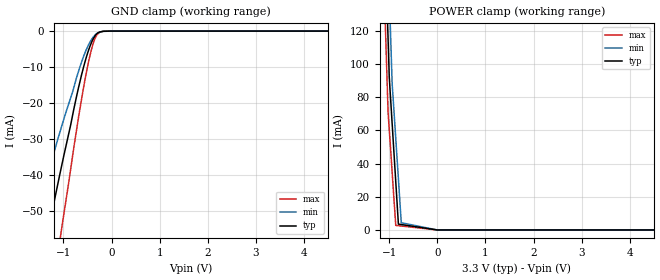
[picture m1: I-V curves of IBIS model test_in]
|DESCRIPTION OF BUG:
|Placing multiple decimal points in sequence in an IBIS file [Package]
|section causes the IBIS parser to "crash" or end execution abruptly.
|The "crash" does not occur if repeated decimal points are present in
|sections other than under the [Package] keyword.
|The parser should flag the repeated decimal points as a simple syntax
|error.
|This problem also occurs in earlier parser versions.
[IBIS Ver]   3.2
[File name]   bug59.ibs
[File rev]   1.0
[Date]   08/01/01
[Source]   From silicon level SPICE model at Intel Corporation.
[Notes]   The following information is for demo purposes only.
[Disclaimer] This IBIS model is provided in connection with Intel
   products. No license, express or implied, by estoppel or
   otherwise, to any intellectual property rights is granted
   by this document. Except as provided in Intel's Terms and
   Conditions of Sale for such products, Intel assumes no
   liability whatsoever, and Intel disclaims any express or
   implied warranty, relating to sale and/or use of Intel
   products including liability or warranties relating to
   fitness for a particular purpose, merchantability, or
   infringement of any patent, copyright or other
   intellectual property right. Intel products are not
   intended for use in medical, life saving, or life
   sustaining applications.
[Copyright]   Copyright 2001, Intel Corporation, All Rights Reserved.
[Component]   TEST
[Manufacturer]  Intel Corporation
[Package]
|   typ   min   max
R_pkg   0mOhm   0mOhm   0mOhm
L_pkg   0.00nH   0.00nH   0.00nH
C_pkg   0..00pF   0.00pF   0.00pF
[Pin]   signal_name   model_name   R_pin   L_pin   C_pin
1   TEST_IN   test_in
| Models and submodels in the file (1): test_in (Input)
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[Model]   test_in
Model_type   Input
Vinl = 0.8V
Vinh = 2.0V
|   typ   min   max
C_comp   3.11pF   2.69pF   3.33pF
[Voltage Range]   3.300V   3.135V   3.465V
[Temperature Range]   25.0   100.0   0.0
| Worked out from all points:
|   GND clamp passes 1 mA (typ) near -0.32 V on its own axis
[GND Clamp]
|   Voltage   I(typ)   I(min)   I(max)
-3.3V     -203.8mA   -150.7mA   -277.6mA
-1.725V   -84.17mA   NA         NA
-1.54V    -71.04mA   NA         NA
-1.33V    -56.54mA   NA         NA
-1.08V    -40.1mA    NA         NA
-995mV    -34.78mA   NA         NA
-695mV    -16.2mA    NA         NA
-495mV    -6.008mA   NA         NA
-375mV    -2.013mA   NA         NA
-315mV    -878.5uA   NA         NA
-250mV    -273.8uA   NA         NA
6.595V    0A         0A         0A
[POWER Clamp]
|   Voltage   I(typ)   I(min)   I(max)
-3.3V     2.388A     2.407A     2.381A
-2.055V   1.081A     NA         NA
-1V       92.25mA    NA         NA
-810mV    3.539mA    NA         NA
0V        1.5uA      2.325uA    1.572uA
6.595V    0A         0A         0A
